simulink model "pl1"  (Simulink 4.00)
settings: Solver=ode45  StartTime=0.0  StopTime=8  RelTol=1e-3

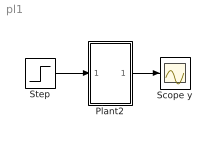
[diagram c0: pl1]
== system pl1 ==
  Plant2 : Subsystem
  Scope y : Scope
  Step : Step  Time=0  Before=0  After=1  SampleTime=0
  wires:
  Step/1 -> Plant2/1(u)
  Plant2/1(y) -> Scope y/1

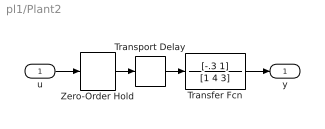
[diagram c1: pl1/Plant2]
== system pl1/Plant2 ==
  u : Inport  Port=1  LatchInput=off
  Transfer Fcn : TransferFcn  Numerator=[-.3 1]  Denominator=[1 4 3]  AbsoluteTolerance=auto  Realization=auto
  Transport Delay : TransportDelay  DelayTime=.2  InitialInput=0  BufferSize=1024  PadeOrder=0
  Zero-Order Hold : ZeroOrderHold  SampleTime=0.1
  y : Outport  Port=1
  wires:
  Zero-Order Hold/1 -> Transport Delay/1
  Transport Delay/1 -> Transfer Fcn/1
  u/1 -> Zero-Order Hold/1
  Transfer Fcn/1 -> y/1
